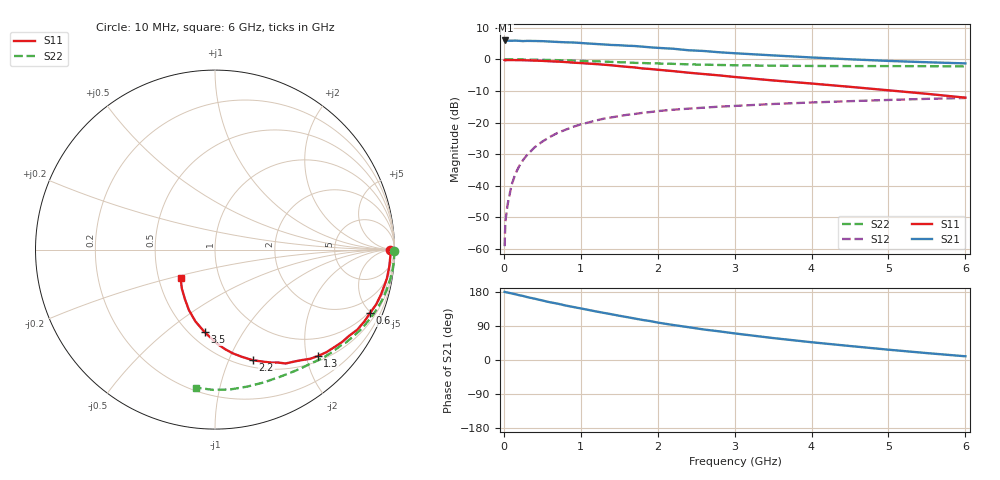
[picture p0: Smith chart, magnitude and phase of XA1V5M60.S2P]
! SIEMENS Discrete & RF Semiconductors
! BFY180
! Si NPN RF Bipolar Junction Transistor in MICRO-X
! VCE = 1.5 V  IC = 0.6 mA
! Common Emitter S-Parameters:  May  1997
# GHz  S  MA  R  50
!  f  S11  S21  S12  S22
! GHz  MAG  ANG  MAG  ANG  MAG  ANG  MAG  ANG
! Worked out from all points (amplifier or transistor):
!   36 points, 10 MHz to 6 GHz, reference 50 ohm
!   highest |S21| = 6.0 dB at 20 MHz (marker M1)
!   |S21| within 3 dB of that: start of sweep to 2.357 GHz
!   unconditionally stable (mu >= 1): 4.395 GHz to end of sweep
!   at 250 MHz: K = 0.06, MSG = 18.8 dB, |S12| = -31.9 dB
!   at 1.4 GHz: K = 0.44, MSG = 11.5 dB, |S12| = -18.4 dB
!   at 6 GHz: K = 1.05, MAG = 4.1 dB, |S12| = -12.2 dB
!   S11 on the Smith chart (normalised r, x): 10 MHz: 86, -13; 600 MHz: 0.89, -4.94; 1.3 GHz: 0.60, -2.22; 2.2 GHz: 0.57, -1.23; 3.5 GHz: 0.59, -0.69; 6 GHz: 0.65, -0.22
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0.01  0.9776 -0.2  1.967 179.9  0.0011 92.9  0.9992 -0.3
0.02  0.967 -0.6  1.997 179.1  0.0027 102.4  0.9999 -0.5
0.05  0.9782 -1.7  1.979 177.9  0.0051 89.6  0.9982 -1.2
0.1  0.9765 -3.7  1.975 175.7  0.0102 88.4  0.9988 -2.5
0.15  0.9755 -5.8  1.985 173.5  0.0154 85.8  0.9996 -3.7
0.2  0.9729 -7.4  1.971 171.0  0.0204 84.5  0.9972 -4.9
0.3  0.9665 -11.3  1.966 166.2  0.0304 81.5  0.9929 -7.2
0.4  0.9582 -15.1  1.958 161.8  0.0405 78.9  0.9906 -9.7
0.6  0.9339 -22.2  1.919 152.3  0.0592 73.2  0.9795 -14.4
0.9  0.8884 -32.7  1.855 140.0  0.0854 65.1  0.9564 -21.3
1.1  0.8591 -39.2  1.785 132.1  0.1003 60.2  0.9391 -25.5
1.3  0.8248 -46.0  1.726 124.4  0.1152 55.6  0.9223 -29.5
1.7  0.7467 -58.2  1.631 109.5  0.1366 47.6  0.8823 -37.0
2  0.6862 -65.8  1.525 98.8  0.1518 42.5  0.8633 -42.1
2.2  0.6525 -71.0  1.477 92.4  0.1597 39.0  0.8509 -45.4
2.6  0.5863 -80.3  1.36 80.5  0.1722 33.7  0.825 -51.2
3  0.5272 -88.3  1.253 70.2  0.1833 28.8  0.8087 -56.9
3.5  0.4646 -97.0  1.158 57.9  0.1967 23.8  0.7953 -63.3
4  0.415 -105.2  1.074 46.9  0.2079 18.9  0.7881 -70.0
4.5  0.3678 -113.2  1.004 36.9  0.2181 14.6  0.7842 -76.7
5.5  0.2851 -130.4  0.902 18.2  0.2373 5.7  0.7816 -90.7
6  0.2477 -140.8  0.865 9.8  0.2448 1.3  0.7763 -97.7
